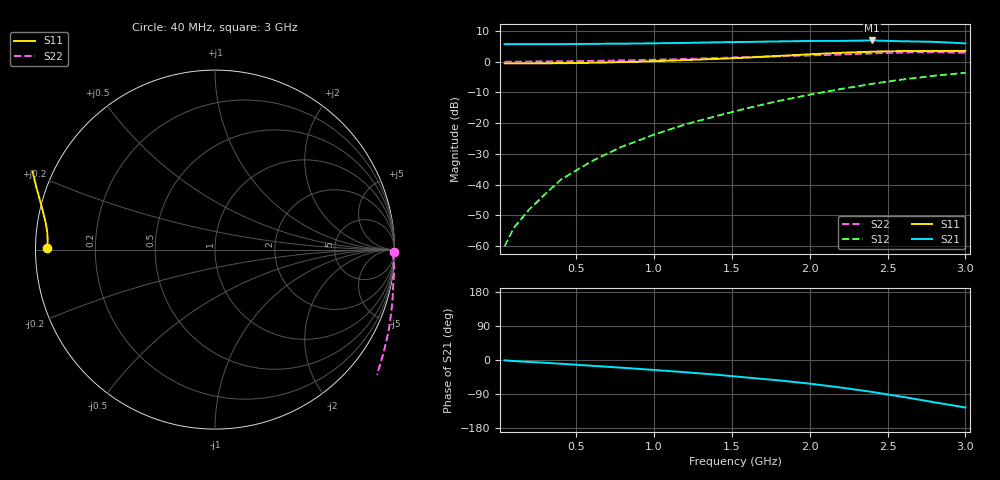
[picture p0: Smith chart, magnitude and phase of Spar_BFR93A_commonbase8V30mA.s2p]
! Filename:  BFR93ACH.S2P  Version:  2.0
! NXP part #: BFR93A  Date: Jul 1990
! Bias condition: Vce=8V, Ic=30mA
! COMMON BASE
#  MHz  S  MA  R  50
! Freq  S11  S21  S12  S22
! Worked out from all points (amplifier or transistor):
!   21 points, 40 MHz to 3 GHz, reference 50 ohm
!   highest |S21| = 6.9 dB at 2.4 GHz (marker M1)
!   |S21| within 3 dB of that: start of sweep to end of sweep
!   unconditionally stable (mu >= 1): nowhere
!   at 300 MHz: K = -0.60, MSG = 24.4 dB, |S12| = -43.1 dB
!   at 1 GHz: K = -0.93, MSG = 14.8 dB, |S12| = -23.7 dB
!   at 3 GHz: K = -0.85, MSG = 4.8 dB, |S12| = -3.6 dB
40  0.934 179.4  1.919 -0.9  0.001 51.8  0.995 -0.8
100  0.933 178.2  1.918 -2.8  0.002 80.8  0.994 -2.6
200  0.934 176.7  1.922 -5.1  0.004 105.9  0.999 -4.7
300  0.937 175.2  1.92 -7.4  0.007 121.6  1.006 -7.1
400  0.941 173.7  1.921 -9.9  0.012 130.8  1.009 -9.7
500  0.948 172.3  1.932 -12.6  0.017 135.5  1.015 -12.2
600  0.957 170.7  1.938 -15.2  0.024 140.0  1.024 -14.8
700  0.969 169.1  1.949 -17.9  0.032 141.4  1.034 -17.4
800  0.982 167.5  1.955 -20.5  0.042 143.2  1.044 -20.1
900  0.997 165.8  1.966 -23.4  0.052 143.8  1.056 -22.7
1000  1.015 164.1  1.982 -26.3  0.065 143.9  1.07 -25.5
1200  1.056 160.6  2.009 -32.2  0.095 143.0  1.101 -31.4
1400  1.106 156.8  2.057 -38.8  0.13 140.5  1.141 -37.7
1600  1.162 152.6  2.087 -46.3  0.175 138.1  1.182 -44.5
1800  1.235 147.7  2.126 -53.7  0.229 133.8  1.22 -52.1
2000  1.312 142.4  2.164 -62.4  0.29 128.7  1.26 -60.7
2200  1.39 136.8  2.167 -72.7  0.358 122.8  1.302 -71.1
2400  1.449 129.9  2.204 -84.2  0.434 115.4  1.36 -82.3
2600  1.481 122.0  2.137 -97.5  0.513 107.4  1.406 -93.6
2800  1.486 112.3  2.092 -111.5  0.588 98.4  1.422 -105.2
3000  1.489 102.6  1.976 -125.5  0.657 90.4  1.395 -116.8
